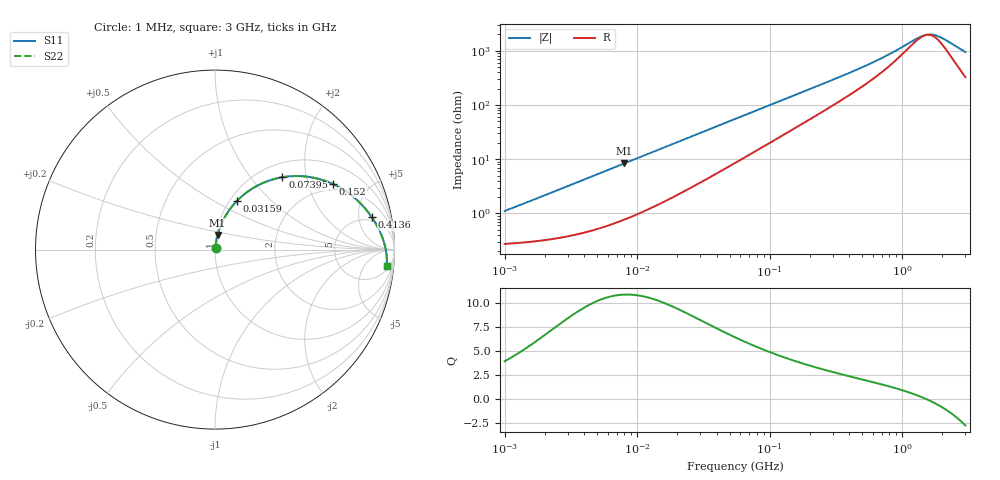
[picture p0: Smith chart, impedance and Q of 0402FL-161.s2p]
# MHz S MA R 50
!Freq  MagS11  AngS11  MagS21  AngS21  MagS12  AngS12  MagS22  AngS22
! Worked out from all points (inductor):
!   801 points, 1 MHz to 3 GHz, reference 50 ohm
!   read as one part in series: L = 170 nH near 1.041 MHz
!   highest Q = 10.8 at 8.018 MHz (marker M1), where L = 166 nH
!   self-resonance near 1.52 GHz
!   S11 on the Smith chart (normalised r, x): 1 MHz: 1.01, +0.02; 31.59 MHz: 1.08, +0.64; 73.95 MHz: 1.26, +1.46; 152 MHz: 1.73, +2.90; 413.6 MHz: 4.22, +7.46; 3 GHz: 8, -18
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1  0.01106 75.1  0.9972 -0.6  0.9972 -0.6  0.01106 75.1
3.823119  0.04033 81.6  0.9949 -2.3  0.9949 -2.3  0.04033 81.6
8.017732  0.08296 80.0  0.989 -4.7  0.989 -4.7  0.08296 80.0
14.47069  0.1461 76.0  0.9751 -8.4  0.9751 -8.4  0.1461 76.0
22.0312  0.2158 71.4  0.9532 -12.4  0.9532 -12.4  0.2158 71.4
31.58701  0.2963 65.8  0.9192 -17.1  0.9192 -17.1  0.2963 65.8
41.80303  0.3725 60.4  0.8782 -21.6  0.8782 -21.6  0.3725 60.4
54.77226  0.4548 54.4  0.8233 -26.7  0.8233 -26.7  0.4548 54.4
73.95247  0.5508 47.1  0.7436 -32.8  0.7436 -32.8  0.5508 47.1
104.9728  0.6574 38.1  0.6307 -40.1  0.6307 -40.1  0.6574 38.1
152.0175  0.7513 29.2  0.5022 -46.8  0.5022 -46.8  0.7513 29.2
209.4008  0.8126 22.4  0.3969 -51.2  0.3969 -51.2  0.8126 22.4
288.4452  0.8573 16.7  0.3048 -54.0  0.3048 -54.0  0.8573 16.7
413.5554  0.8923 11.6  0.2197 -55.0  0.2197 -55.0  0.8923 11.6
587.0266  0.9159 7.7  0.1541 -53.1  0.1541 -53.1  0.9159 7.7
792.5923  0.9307 5.0  0.1089 -48.0  0.1089 -48.0  0.9307 5.0
1333.714  0.9484 1.0  0.05411 -17.1  0.05411 -17.1  0.9484 1.0
1474.099  0.9509 0.2  0.04923 -4.4  0.04923 -4.4  0.9509 0.2
1613.037  0.953 -0.4  0.04762 8.8  0.04762 8.8  0.953 -0.4
1765.07  0.9548 -1.1  0.04897 22.1  0.04897 22.1  0.9548 -1.1
1950.859  0.9566 -1.9  0.05382 35.3  0.05382 35.3  0.9566 -1.9
3000  0.9607 -5.5  0.1013 64.5  0.1013 64.5  0.9607 -5.5
